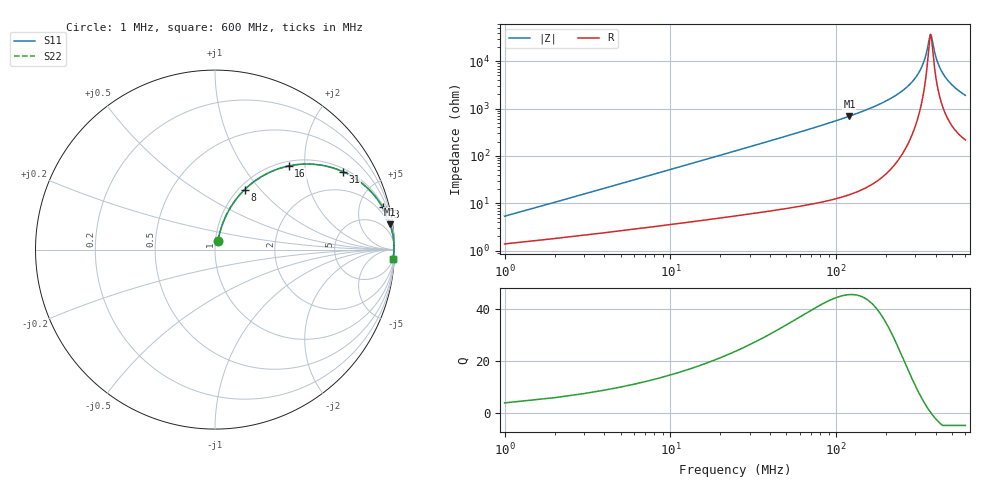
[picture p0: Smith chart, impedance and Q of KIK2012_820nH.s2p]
!version-2
!date-01.2022
!Series
# MHz S RI R 50
!Freq ReS11 ImS11 ReS21 ImS21 ReS12 ImS12 ReS22 ImS22
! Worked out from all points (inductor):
!   600 points, 1 MHz to 600 MHz, reference 50 ohm
!   read as one part in series: L = 820 nH near 4 MHz
!   highest Q = 45.6 at 120 MHz (marker M1), where L = 916 nH
!   self-resonance near 370 MHz
!   S11 on the Smith chart (normalised r, x): 1 MHz: 1.03, +0.10; 8 MHz: 1.06, +0.82; 16 MHz: 1.09, +1.65; 31 MHz: 1.12, +3.22; 73 MHz: 1.20, +7.83; 600 MHz: 5, -38
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1  0.0162 0.05  0.9838 -0.05  0.9838 -0.05  0.0162 0.05
5  0.0833 0.2302  0.9167 -0.2302  0.9167 -0.2302  0.0833 0.2302
8  0.1645 0.3338  0.8355 -0.3338  0.8355 -0.3338  0.1645 0.3338
12  0.2895 0.4234  0.7105 -0.4234  0.7105 -0.4234  0.2895 0.4234
16  0.4108 0.4661  0.5892 -0.4661  0.5892 -0.4661  0.4108 0.4661
31  0.7143 0.4334  0.2857 -0.4334  0.2857 -0.4334  0.7143 0.4334
48  0.8563 0.3361  0.1437 -0.3361  0.1437 -0.3361  0.8563 0.3361
73  0.9335 0.2369  0.0665 -0.2369  0.0665 -0.2369  0.9335 0.2369
101  0.9657 0.171  0.0343 -0.171  0.0343 -0.171  0.9657 0.171
120  0.9765 0.1409  0.0235 -0.1409  0.0235 -0.1409  0.9765 0.1409
201  0.9934 0.0675  0.00657 -0.0675  0.00657 -0.0675  0.9934 0.0675
260  0.9966 0.0377  0.00341 -0.0377  0.00341 -0.0377  0.9966 0.0377
301  0.9974 0.0218  0.00265 -0.0218  0.00265 -0.0218  0.9974 0.0218
338  0.9975 0.00958  0.00252 -0.00958  0.00252 -0.00958  0.9975 0.00958
369  0.9973 0.000431  0.0027 -0.000431  0.0027 -0.000431  0.9973 0.000431
375  0.9972 -0.00125  0.00276 0.00125  0.00276 0.00125  0.9972 -0.00125
389  0.9971 -0.00506  0.00293 0.00506  0.00293 0.00506  0.9971 -0.00506
401  0.9969 -0.00822  0.0031 0.00822  0.0031 0.00822  0.9969 -0.00822
418  0.9966 -0.0125  0.00339 0.0125  0.00339 0.0125  0.9966 -0.0125
440  0.9962 -0.0179  0.00382 0.0179  0.00382 0.0179  0.9962 -0.0179
501  0.9947 -0.0317  0.00534 0.0317  0.00534 0.0317  0.9947 -0.0317
600  0.9913 -0.0515  0.00865 0.0515  0.00865 0.0515  0.9913 -0.0515
